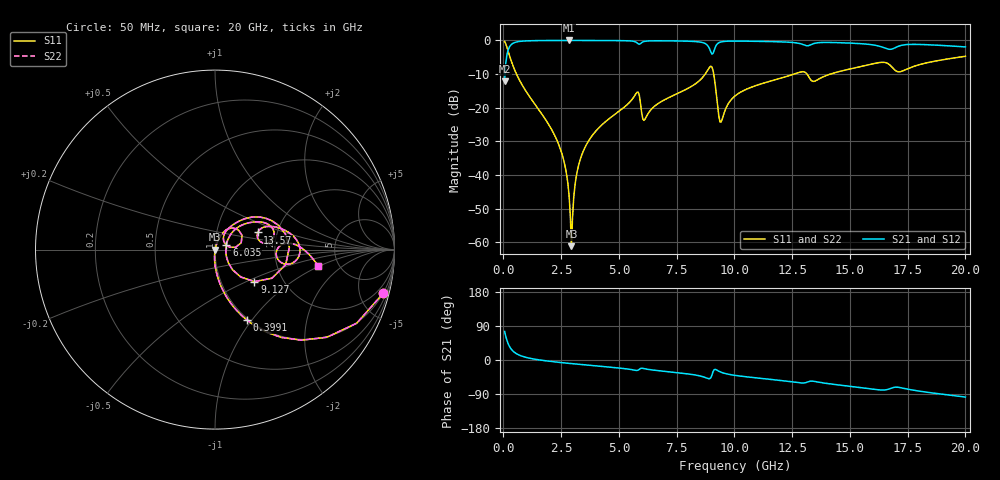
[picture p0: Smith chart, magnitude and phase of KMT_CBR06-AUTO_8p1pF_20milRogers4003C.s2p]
! Data measured by Modelithics Inc. support@modelithics.com 813-866-6335
! KEMET CBR06-AUTO 8.1pF, Pad Width= 0.851mm, Pad Length= 0.64mm, Pad Gap= 0.62mm, 20mil Rogers 4003C substrate Data, January 2022
# hz S ma R 50
! 2 Port Network Data from SP1.SP block
! freq  magS11  angS11  magS21  angS21  magS12  angS12  magS22  angS22
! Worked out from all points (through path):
!   401 points, 50 MHz to 20 GHz, reference 50 ohm
!   highest |S21| = -0.01 dB at 2.843 GHz (marker M1); lowest = -12.1 dB at 50 MHz (marker M2)
!   group delay of S21, straight-line fit = 14.6 ps
!   lowest |S11| = -61.1 dB at 2.943 GHz (marker M3), VSWR 1.00, Z = 50.1 - j0.0221 ohm
!   |S11| at or under -10 dB: 564.5 MHz to 8.734 GHz (8.169 GHz wide, 176 % of centre); 9.103 GHz to 12.58 GHz (3.479 GHz wide, 32.1 % of centre); 13.14 GHz to 14.15 GHz (1.008 GHz wide, 7.38 % of centre)
!   |S22| runs from -61.1 to -0.3 dB; largest |S21 - S12| = 0
!   S11 on the Smith chart (normalised r, x): 50 MHz: 0.98, -7.72; 399.1 MHz: 0.98, -0.95; 6.035 GHz: 1.13, +0.06; 9.127 GHz: 1.44, -0.56; 13.57 GHz: 1.59, +0.32; 20 GHz: 3.49, -0.97
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5e7  0.9686 -14.5  0.2483 75.4  0.2483 75.4  0.9686 -14.5
3.99125e8  0.4326 -65.6  0.901 24.3  0.901 24.3  0.4326 -65.6
2.34425e9  0.03123 -94.3  0.9986 -5.8  0.9986 -5.8  0.03123 -94.3
2.693375e9  0.01226 -94.1  0.999 -8.0  0.999 -8.0  0.01226 -94.1
2.843e9  0.004902 -88.8  0.999 -8.9  0.999 -8.9  0.004902 -88.8
2.94275e9  0.0008799 -14.5  0.999 -9.5  0.999 -9.5  0.0008799 -14.5
3.192125e9  0.0113 74.4  0.9989 -10.9  0.9989 -10.9  0.0113 74.4
3.391625e9  0.01994 75.2  0.9987 -12.1  0.9987 -12.1  0.01994 75.2
4.04e9  0.04665 72.9  0.9976 -15.7  0.9976 -15.7  0.04665 72.9
5.73575e9  0.1619 46.8  0.9435 -27.4  0.9435 -27.4  0.1619 46.8
6.035e9  0.06785 21.1  0.9492 -22.1  0.9492 -22.1  0.06785 21.1
6.73325e9  0.1178 59.1  0.9876 -28.4  0.9876 -28.4  0.1178 59.1
8.72825e9  0.3141 35.0  0.9009 -46.0  0.9009 -46.0  0.3141 35.0
8.977625e9  0.4144 1.6  0.6752 -46.7  0.6752 -46.7  0.4144 1.6
9.12725e9  0.2827 -39.1  0.7229 -25.3  0.7229 -25.3  0.2827 -39.1
9.4265e9  0.0615 8.7  0.9525 -32.4  0.9525 -32.4  0.0615 8.7
1.0025e10  0.1496 45.2  0.9775 -40.6  0.9775 -40.6  0.1496 45.2
1.286788e10  0.3399 21.3  0.8926 -60.4  0.8926 -60.4  0.3399 21.3
1.336662e10  0.2487 12.7  0.8806 -55.7  0.8806 -55.7  0.2487 12.7
1.356612e10  0.2568 21.8  0.9196 -57.5  0.9196 -57.5  0.2568 21.8
1.670825e10  0.4383 -9.9  0.7389 -76.1  0.7389 -76.1  0.4383 -9.9
2e10  0.5815 -9.1  0.8001 -97.8  0.8001 -97.8  0.5815 -9.1
